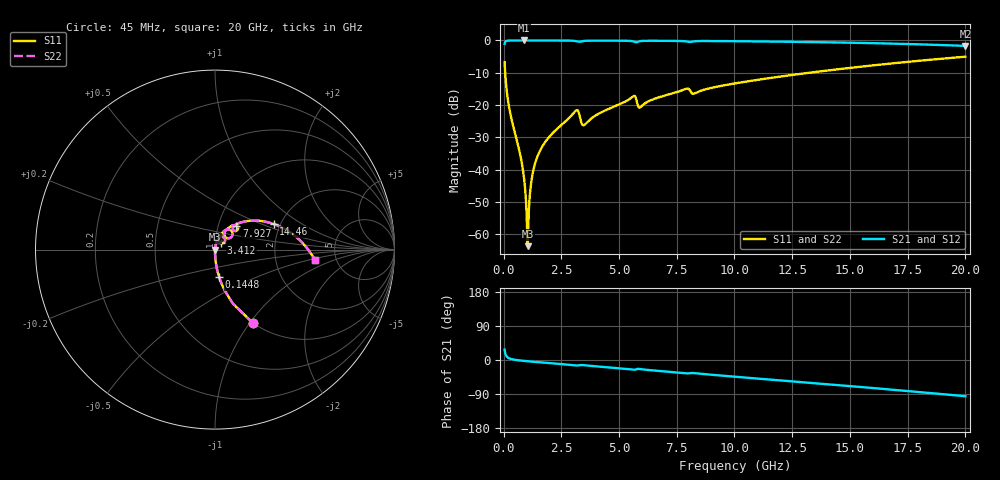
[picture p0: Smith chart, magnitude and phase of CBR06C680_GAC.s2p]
! S-parameter model data by Modelithics Inc.  support@modelithics.com 813-866-6335  Tampa FL USA
! S-Parameter data specifications:
! Substrate: 20-mil Rogers 4350B, substrate thickness, H=0.508mm, Dielectric constant, Er=3.75
! PCB Mounting Pad Footprint: Pad width, PadW=0.85mm , Pad length, PadL=0.64mm , Pad gap, PadG (edge-to-edge)=0.62mm , Reference planes=1.9mm apart
#  GHz  S  MA  R 50
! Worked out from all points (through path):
!   801 points, 45 MHz to 20 GHz, reference 50 ohm
!   highest |S21| = -0.01 dB at 893.1 MHz (marker M1); lowest = -1.7 dB at 20 GHz (marker M2)
!   group delay of S21, straight-line fit = 13.4 ps
!   lowest |S11| = -63.7 dB at 1.043 GHz (marker M3), VSWR 1.00, Z = 50.1 - j0.000896 ohm
!   |S11| at or under -10 dB: 69.77 MHz to 13.24 GHz (13.17 GHz wide, 198 % of centre)
!   |S22| runs from -63.7 to -5.0 dB; largest |S21 - S12| = 0
!   S11 on the Smith chart (normalised r, x): 45 MHz: 1.00, -1.03; 144.8 MHz: 1.00, -0.32; 3.412 GHz: 1.07, +0.08; 7.927 GHz: 1.22, +0.34; 14.46 GHz: 1.85, +0.60; 20 GHz: 3.44, -0.58
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0.045  0.4599 -62.7  0.8876 27.2  0.8876 27.2  0.4599 -62.7
0.144775  0.1563 -81.4  0.9874 8.5  0.9874 8.5  0.1563 -81.4
0.743425  0.0155 -89.4  0.9993 -1.5  0.9993 -1.5  0.0155 -89.4
0.893088  0.007017 -87.5  0.9993 -2.4  0.9993 -2.4  0.007017 -87.5
0.967919  0.003398 -82.2  0.9993 -2.9  0.9993 -2.9  0.003398 -82.2
1.04275  0.000652 -0.8  0.9993 -3.3  0.9993 -3.3  0.000652 -0.8
1.117581  0.003243 74.3  0.9993 -3.7  0.9993 -3.7  0.003243 74.3
1.217356  0.007125 80.1  0.9992 -4.3  0.9992 -4.3  0.007125 80.1
1.317131  0.01079 81.3  0.9991 -4.8  0.9991 -4.8  0.01079 81.3
1.691288  0.02324 81.2  0.9988 -6.7  0.9988 -6.7  0.02324 81.2
3.113081  0.08093 61.6  0.9772 -14.4  0.9772 -14.4  0.08093 61.6
3.387462  0.05164 43.3  0.9705 -13.2  0.9705 -13.2  0.05164 43.3
3.412406  0.04972 46.8  0.9741 -13.3  0.9741 -13.3  0.04972 46.8
5.607456  0.1362 54.8  0.9677 -25.5  0.9677 -25.5  0.1362 54.8
5.906781  0.09152 51.9  0.9732 -23.8  0.9732 -23.8  0.09152 51.9
6.704981  0.1307 59.7  0.9876 -28.7  0.9876 -28.7  0.1307 59.7
7.927225  0.1792 48.5  0.9641 -35.3  0.9641 -35.3  0.1792 48.5
10.0225  0.2161 45.2  0.973 -44.0  0.973 -44.0  0.2161 45.2
13.36496  0.3202 29.1  0.9438 -60.4  0.9438 -60.4  0.3202 29.1
14.46249  0.3572 23.5  0.9303 -66.0  0.9303 -66.0  0.3572 23.5
16.68248  0.4359 12.0  0.8958 -77.6  0.8958 -77.6  0.4359 12.0
20  0.5598 -6.0  0.8237 -95.6  0.8237 -95.6  0.5598 -6.0
